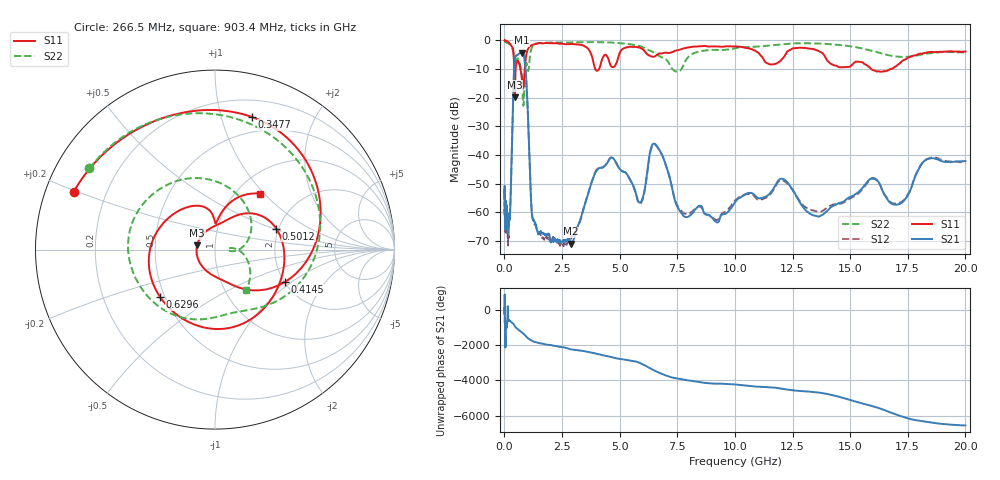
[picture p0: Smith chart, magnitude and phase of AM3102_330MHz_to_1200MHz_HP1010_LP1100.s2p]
! Date/Time: Tue, Sep 11, 2018 5:19 PM
! Network Analyzer: Agilent Technologies E8362B Rev: A.07.50.63
! Sweep from 0.010 to 20.000 GHz, 1601 Points, Sweep Type: LOG
! Power Supply: 4.949 V, 0.001 A
# Hz S DB R 50
!freq MagS11 AngS11 MagS21 AngS21 MagS12 AngS12 MagS22 AngS22
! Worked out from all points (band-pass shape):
!   1601 points, 10 MHz to 20 GHz, reference 50 ohm
!   highest |S21| = -4.25 dB at 761.4 MHz (marker M1); lowest = -70.9 dB at 2.893 GHz (marker M2)
!   |S21| within 3 dB of the highest: 440.6 MHz to 884.5 MHz (443.9 MHz wide, 67 % of centre)
!   lowest |S11| = -19.8 dB at 451.5 MHz (marker M3), VSWR 1.23, Z = 40.9 + j2.03 ohm
!   |S11| at or under -10 dB: 696 MHz to 881.3 MHz (185.3 MHz wide, 23.5 % of centre); 3.949 GHz to 4.106 GHz (156.4 MHz wide, 3.88 % of centre); 15.91 GHz to 16.77 GHz (854.7 MHz wide, 5.23 % of centre)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
!   |S22| runs from -22.8 to -0.2 dB; largest |S21 - S12| = 0.0097
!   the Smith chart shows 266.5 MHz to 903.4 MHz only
!   S11 on the Smith chart (normalised r, x): 266.5 MHz: 0.08, +0.19; 347.7 MHz: 0.35, +1.25; 414.5 MHz: 2.02, -0.89; 501.2 MHz: 1.94, +0.52; 629.6 MHz: 0.47, -0.30; 903.4 MHz: 1.28, +0.95
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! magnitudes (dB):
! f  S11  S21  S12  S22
! 10 MHz  0.0  -52.8  -51.7  -0.2
! 35.55 MHz  0.0  -65.3  -62.9  -0.5
! 126.4 MHz  -0.4  -65.0  -64.7  -0.9
! 266.5 MHz  -1.4  -55.9  -55.6  -1.6
! 347.7 MHz  -2.3  -30.9  -31.0  -2.8
! 414.5 MHz  -7.3  -11.4  -11.4  -6.0
! 447.2 MHz  -19.6  -6.7  -6.7  -8.6
! 451.5 MHz  -19.8  -6.4  -6.5  -8.7
! 501.2 MHz  -8.9  -5.3  -5.4  -7.3
! 629.6 MHz  -7.9  -4.6  -4.8  -6.9
! 761.4 MHz  -13.4  -4.3  -4.3  -13.9
! 903.4 MHz  -7.9  -8.7  -8.7  -10.9
! 1.196 GHz  -1.6  -60.7  -60.3  -2.4
! 1.59 GHz  -1.0  -66.7  -67.9  -0.9
! 2.893 GHz  -1.2  -70.9  -68.9  -0.7
! 4.564 GHz  -7.8  -41.3  -41.2  -0.7
! 5.652 GHz  -2.3  -51.9  -52.2  -1.6
! 6.58 GHz  -5.3  -36.5  -36.7  -4.7
! 7.808 GHz  -2.7  -61.4  -60.4  -7.9
! 12.03 GHz  -6.6  -48.2  -48.7  -1.4
! 13.61 GHz  -3.7  -61.4  -59.6  -1.1
! 20 GHz  -3.9  -42.1  -42.6  -4.2
